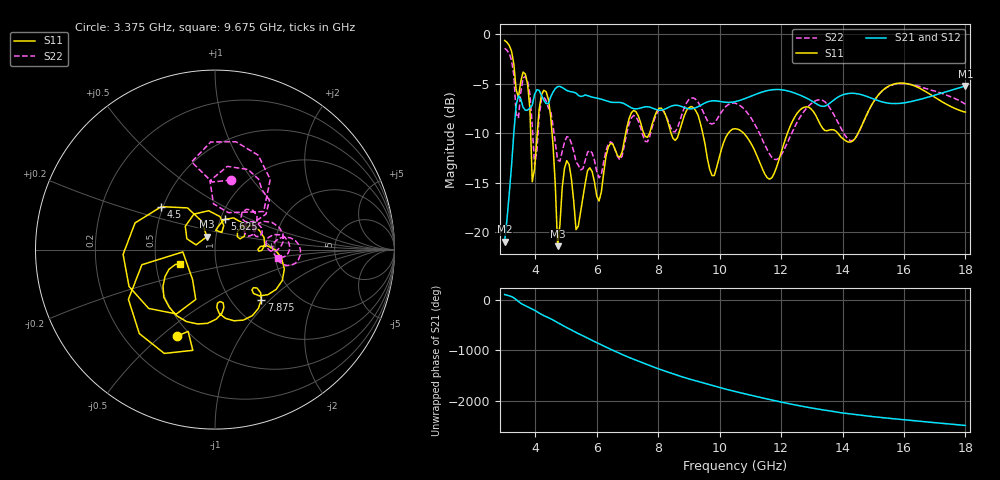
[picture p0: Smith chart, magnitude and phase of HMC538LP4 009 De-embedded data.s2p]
! Chelmsford, MA 01824
! http://www.hittite.com
! Tel: 978-250-3343
! Fax: 978-250-3373
! Device  :  HMC538LP4
! Description:  600 Analog Phase Shifter
! Frequency  :  6.0 GHz - 15.0 GHz
! Package  :  LP4  - 4x4 mm Quad Flatpack No-Lead (QFN) Plastic Package: 24 pin
! Ports  :  2 RF, 1 DC
!  Pin  3  = Rfin  = Port 1
!  Pin  16  = Rfout = Port 2
!  pin  21  = vCTL
! Voltages:  VCTL  = 0 to 5.0 Volts
! Currents :  Vb(V)  Vd(V)  Ib(mA)  Id(mA)
!  0.00  0.90  0.000000	0.482513
! Data:  The device was measured on evaluation board 111296-1.
!  Data was collected using a calibrated network analyzer.
!  The evaluation circuit board was modeled and simulated.This was use
!  to removed the evaluation board circuit from the measured data.
!  The reference plane is the center of the package pin.
! Misc:  Lot #
!Date Measured:  03 - 11 -2009
! Date:  03 - 17 -2009
! Note:
!  Hittite Microwave supplies this data as a sample of measured data at the
!  package pin for this package product.  Your particular data for this product
!  may vary.
!  Data was taken at 25 degrees C.
!  Hittite Microwave reserves the right to change this data at anytime.
# MHz S MA R 50
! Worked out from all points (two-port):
!   201 points, 3 GHz to 18 GHz, reference 50 ohm
!   highest |S21| = -5.22 dB at 18 GHz (marker M1); lowest = -21.0 dB at 3 GHz (marker M2)
!   |S21| within 3 dB of the highest: 3.347 GHz to end of sweep
!   lowest |S11| = -21.4 dB at 4.725 GHz (marker M3), VSWR 1.19, Z = 45.2 + j6.53 ohm
!   |S11| at or under -10 dB: 4.545 GHz to 6.943 GHz (2.398 GHz wide, 41.7 % of centre); 9.451 GHz to 10.28 GHz (831.4 MHz wide, 8.43 % of centre); 10.78 GHz to 12.21 GHz (1.423 GHz wide, 12.4 % of centre)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
!   |S22| runs from -14.5 to -1.4 dB; largest |S21 - S12| = 0.0016
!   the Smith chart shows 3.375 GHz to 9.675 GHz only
!   S11 on the Smith chart (normalised r, x): 3.375 GHz: 0.43, -0.57; 4.5 GHz: 0.49, +0.27; 5.625 GHz: 1.05, +0.36; 7.875 GHz: 1.35, -0.89; 9.675 GHz: 0.67, -0.11
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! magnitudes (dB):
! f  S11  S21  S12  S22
! 3 GHz  -0.6  -21.0  -21.0  -1.4
! 3.375 GHz  -5.6  -7.2  -7.2  -8.0
! 3.75 GHz  -5.1  -7.7  -7.7  -4.8
! 3.9 GHz  -14.9  -7.2  -7.2  -9.3
! 3.975 GHz  -13.6  -6.1  -6.1  -13.2
! 4.2 GHz  -6.1  -6.2  -6.2  -6.6
! 4.5 GHz  -8.3  -6.3  -6.3  -7.8
! 4.725 GHz  -21.4  -5.3  -5.3  -12.7
! 5.025 GHz  -12.8  -5.7  -5.7  -10.3
! 5.325 GHz  -19.7  -5.9  -5.9  -12.9
! 5.55 GHz  -16.5  -6.2  -6.3  -13.6
! 5.625 GHz  -15.0  -6.1  -6.1  -12.8
! 7.875 GHz  -8.4  -7.5  -7.5  -8.6
! 8.025 GHz  -7.5  -7.7  -7.7  -7.7
! 9.15 GHz  -7.4  -7.5  -7.5  -6.4
! 9.675 GHz  -13.6  -6.8  -6.8  -9.0
! 10.5 GHz  -9.5  -6.8  -6.8  -7.0
! 11.62 GHz  -14.6  -5.6  -5.7  -12.1
! 13.05 GHz  -7.8  -6.8  -6.8  -6.9
! 14.32 GHz  -10.8  -6.0  -6.0  -10.7
! 15.53 GHz  -5.2  -7.0  -7.0  -5.2
! 18 GHz  -7.9  -5.2  -5.2  -7.1
